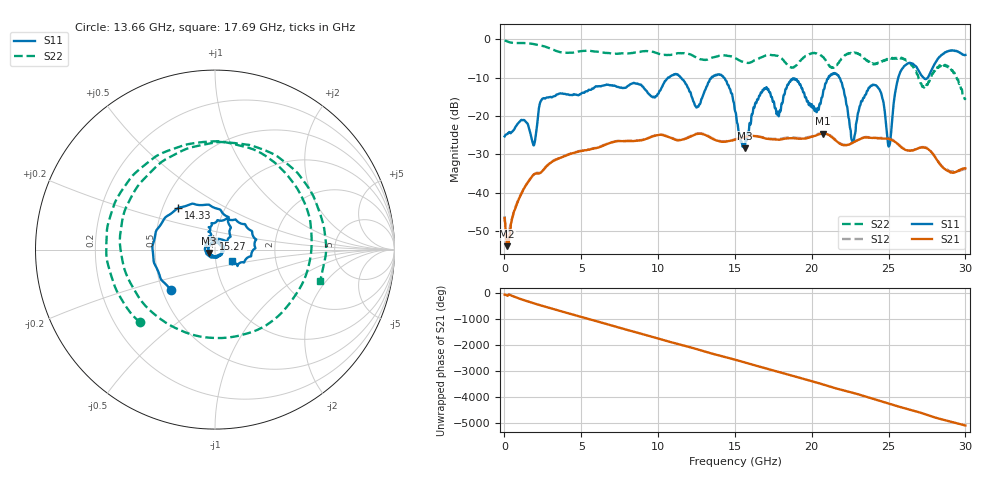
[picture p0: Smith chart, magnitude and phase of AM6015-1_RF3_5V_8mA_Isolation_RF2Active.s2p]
!Agilent Technologies,E8364B,MY43040894,A.07.50.67
!Agilent E8364B: A.07.50.67
!Date: Monday, August 13, 2018 07:06:10
!Correction: S11(Full 2 Port(1,2))
!S21(Full 2 Port(1,2))
!S12(Full 2 Port(1,2))
!S22(Full 2 Port(1,2))
!S2P File: Measurements: S11, S21, S12, S22:
# Hz S  dB  R 50
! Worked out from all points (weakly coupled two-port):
!   1601 points, 10 MHz to 30 GHz, reference 50 ohm
!   highest |S21| = -24.58 dB at 20.72 GHz (marker M1); lowest = -53.9 dB at 178.7 MHz (marker M2)
!   lowest |S11| = -28.4 dB at 15.62 GHz (marker M3), VSWR 1.08, Z = 46.8 - j1.83 ohm
!   |S11| at or under -10 dB: start of sweep to 10.65 GHz; 14.27 GHz to 21.09 GHz (6.823 GHz wide, 38.6 % of centre); 21.79 GHz to 25.63 GHz (3.844 GHz wide, 16.2 % of centre)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
!   |S22| runs from -15.6 to -0.3 dB; largest |S21 - S12| = 0.0063
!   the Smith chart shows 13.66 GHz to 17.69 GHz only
!   S11 on the Smith chart (normalised r, x): 13.66 GHz: 0.55, -0.28; 14.33 GHz: 0.60, +0.31; 15.27 GHz: 0.97, +0.12; 17.69 GHz: 1.19, -0.16
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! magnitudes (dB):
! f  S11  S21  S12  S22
! 10 MHz  -25.3  -46.6  -46.1  -0.3
! 178.7 MHz  -24.7  -53.9  -52.9  -0.6
! 1.809 GHz  -26.5  -35.7  -35.7  -1.2
! 2.465 GHz  -15.5  -34.3  -34.3  -1.7
! 5.015 GHz  -14.1  -29.1  -29.0  -3.1
! 10.02 GHz  -14.2  -24.9  -24.8  -3.8
! 13.66 GHz  -9.5  -26.2  -26.0  -4.7
! 14.33 GHz  -10.2  -26.7  -26.6  -4.2
! 15.01 GHz  -18.6  -26.2  -26.1  -4.9
! 15.27 GHz  -24.4  -25.9  -25.8  -5.5
! 15.62 GHz  -28.4  -25.5  -25.4  -6.0
! 16.82 GHz  -13.2  -25.7  -25.6  -4.6
! 17.69 GHz  -18.9  -26.2  -26.0  -4.3
! 18.79 GHz  -10.2  -25.8  -25.6  -7.4
! 20.01 GHz  -16.9  -25.4  -25.3  -3.7
! 20.72 GHz  -14.3  -24.6  -24.5  -4.6
! 21.73 GHz  -9.5  -26.9  -26.8  -6.2
! 22.69 GHz  -26.4  -26.9  -26.8  -3.6
! 24.19 GHz  -12.0  -25.7  -25.7  -6.3
! 25.01 GHz  -28.0  -25.9  -25.9  -5.0
! 25.99 GHz  -7.1  -28.6  -28.5  -5.2
! 30 GHz  -4.1  -33.7  -33.9  -15.4
